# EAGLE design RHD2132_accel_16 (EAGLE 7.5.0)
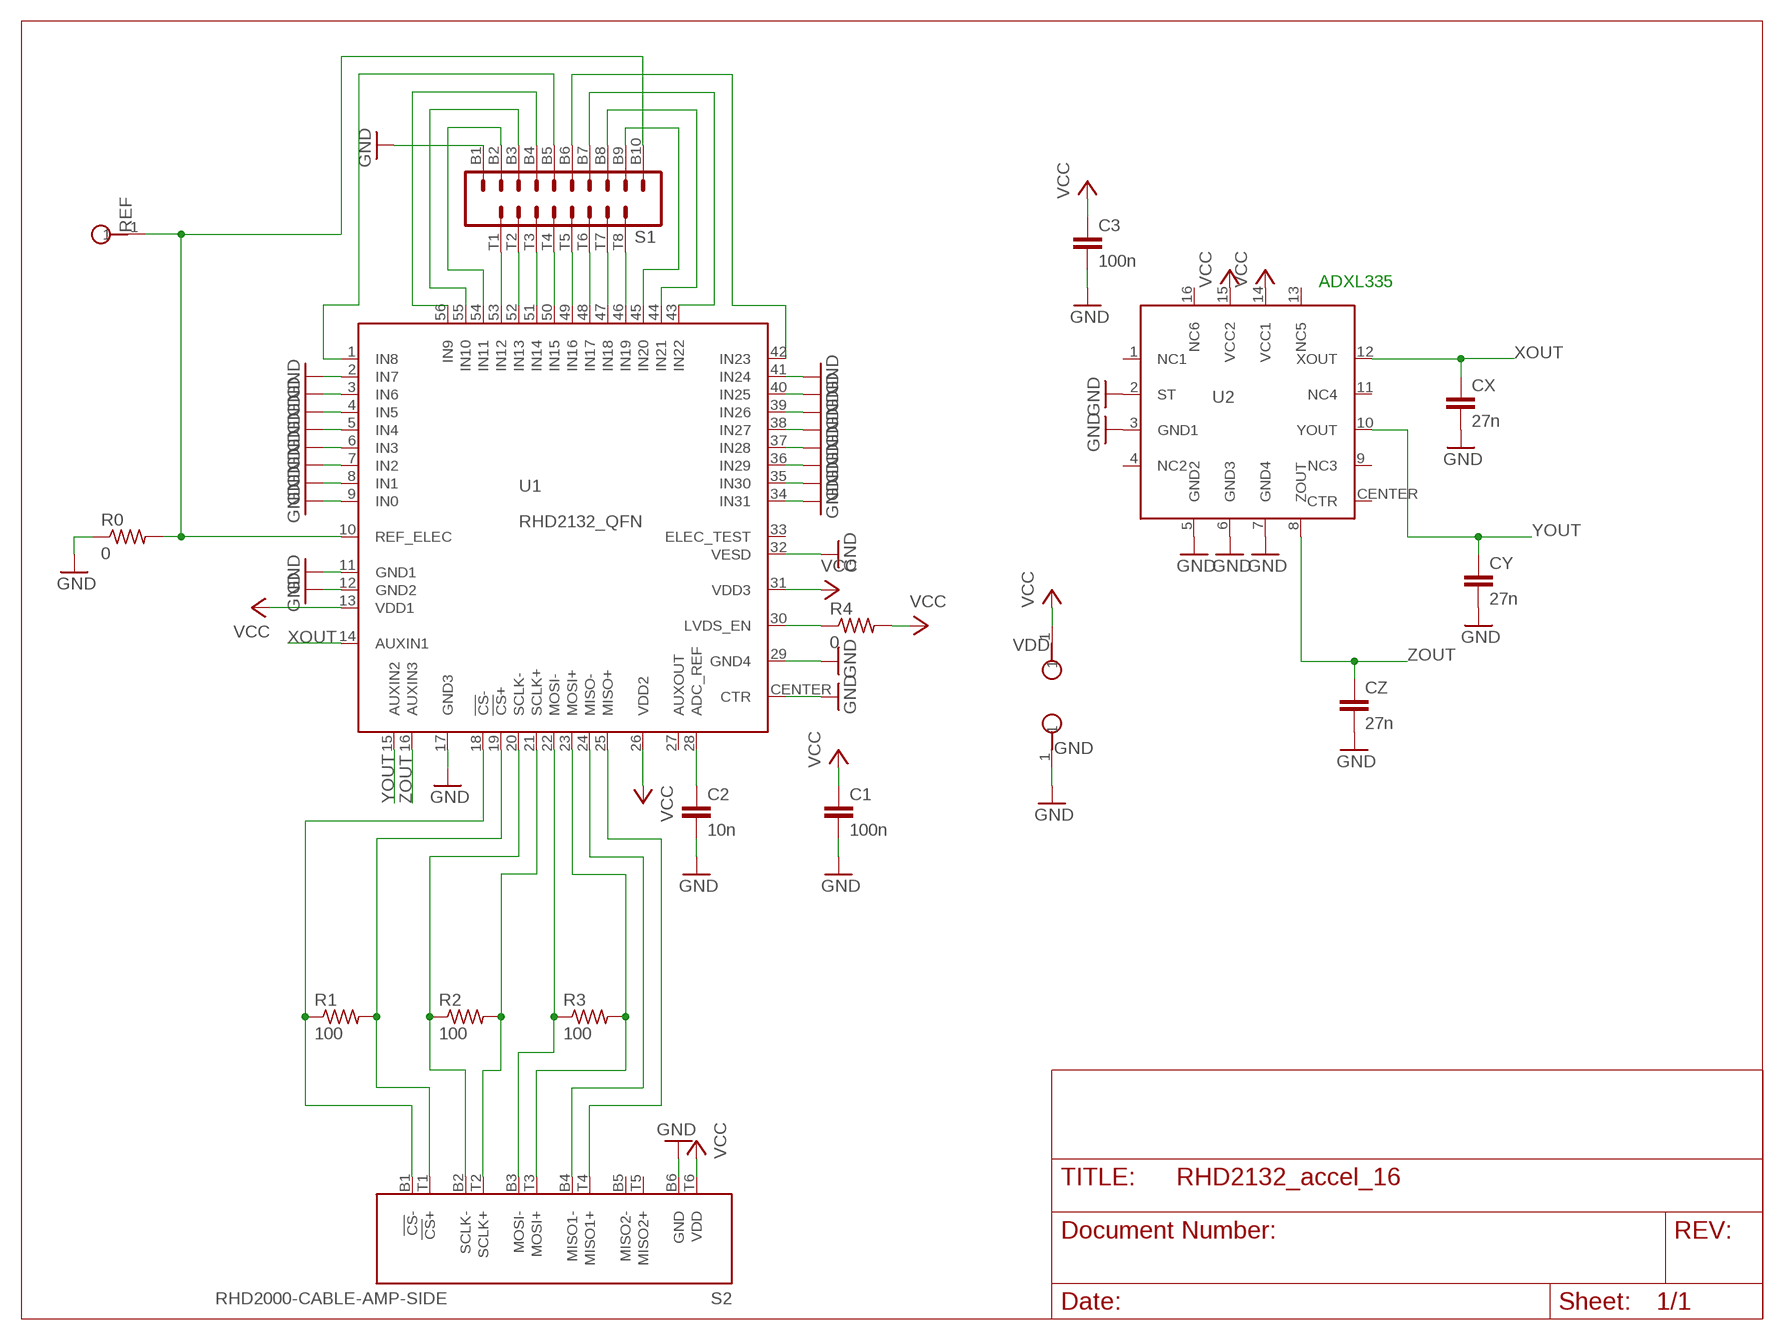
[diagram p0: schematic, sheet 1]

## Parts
C1  100n  C_0402  [0402]
C2  10n  C_0402  [0402]
C3  100n  C_0402  [0402]
CX  27n  C_0402  [0402]
CY  27n  C_0402  [0402]
CZ  27n  C_0402  [0402]
GND  TESTPOINT_SMALL  [TESTPOINT_SMALL]
R0  0  R_0402  [0402]
R1  100  R_0402  [0402]
R2  100  R_0402  [0402]
R3  100  R_0402  [0402]
R4  0  R_0402  [0402]
REF  TESTPOINT_SMALL  [TESTPOINT_SMALL]
S1  OMNETICS_A79041  [OMNETICS_A79041]
S2  RHD2000-CABLE-AMP-SIDE  [OMNETICS_PZN-12-AA]
U1  RHD2132_QFN  [QFN56_8_X_8_LARGE]
U2  ADXL335  [ADXL335]
VDD  TESTPOINT_SMALL  [TESTPOINT_SMALL]

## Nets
GND: C1.2 C2.2 C3.2 CX.2 CY.2 CZ.2 GND.1 R0.1 S1.B1 S2.B6(GND) U1.2(IN7) U1.3(IN6) U1.4(IN5) U1.5(IN4) U1.6(IN3) U1.7(IN2) U1.8(IN1) U1.9(IN0) U1.11(GND1) U1.12(GND2) U1.17(GND3) U1.29(GND4) U1.32(VESD) U1.34(IN31) U1.35(IN30) U1.36(IN29) U1.37(IN28) U1.38(IN27) U1.39(IN26) U1.40(IN25) U1.41(IN24) U1.CENTER(CTR) U2.2(ST) U2.3(GND1) U2.5(GND2) U2.6(GND3) U2.7(GND4)
N$1: R0.2 REF.1 S1.B10 U1.10(REF_ELEC)
N$2: S1.B5 U1.1(IN8)
N$3: S1.B4 U1.56(IN9)
N$4: S1.B3 U1.55(IN10)
N$5: S1.B2 U1.54(IN11)
N$6: S1.T1 U1.53(IN12)
N$7: S1.T2 U1.52(IN13)
N$8: S1.T3 U1.51(IN14)
N$9: S1.T4 U1.50(IN15)
N$10: S1.T5 U1.49(IN16)
N$11: R1.2 S2.T1(!CS!+) U1.19(!CS!+)
N$12: R4.1 U1.30(LVDS_EN)
N$13: S1.T6 U1.48(IN17)
N$14: S1.T7 U1.47(IN18)
N$15: S1.T8 U1.46(IN19)
N$16: S1.B9 U1.45(IN20)
N$17: S1.B8 U1.44(IN21)
N$18: S1.B7 U1.43(IN22)
N$19: S1.B6 U1.42(IN23)
N$21: R1.1 S2.B1(!CS!-) U1.18(!CS!-)
N$22: R2.1 S2.B2(SCLK-) U1.20(SCLK-)
N$37: R2.2 S2.T2(SCLK+) U1.21(SCLK+)
N$38: R3.1 S2.B3(MOSI-) U1.22(MOSI-)
N$39: R3.2 S2.T3(MOSI+) U1.23(MOSI+)
N$40: S2.B4(MISO1-) U1.24(MISO-)
N$41: S2.T4(MISO1+) U1.25(MISO+)
N$42: C2.1 U1.28(ADC_REF)
VCC: C1.1 C3.1 R4.2 S2.T6(VDD) U1.13(VDD1) U1.26(VDD2) U1.31(VDD3) U2.14(VCC1) U2.15(VCC2) VDD.1
XOUT: CX.1 U1.14(AUXIN1) U2.12(XOUT)
YOUT: CY.1 U1.15(AUXIN2) U2.10(YOUT)
ZOUT: CZ.1 U1.16(AUXIN3) U2.8(ZOUT)
Unconnected: S2.B5(MISO2-) S2.T5(MISO2+) U1.27(AUXOUT) U1.33(ELEC_TEST) U2.1(NC1) U2.4(NC2) U2.9(NC3) U2.11(NC4) U2.13(NC5) U2.16(NC6) U2.CENTER(CTR)

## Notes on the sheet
- ADXL335

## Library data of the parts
C1-C3 CX CY CZ = RHD2000_eval_board:C: Capacitor
GND REF VDD = RHD2000_eval_board:TESTPOINT: PCB Test Point
R0 R1-R4 = RHD2000_eval_board:R: Resistor
S1 = harrison:OMNETICS_A79041
S2 = RHD2000:RHD2000-CABLE-AMP-SIDE
U1 = INTAN:RHD2132: Intan Technologies RHD2132 chip
U2 = harrison:ADXL335

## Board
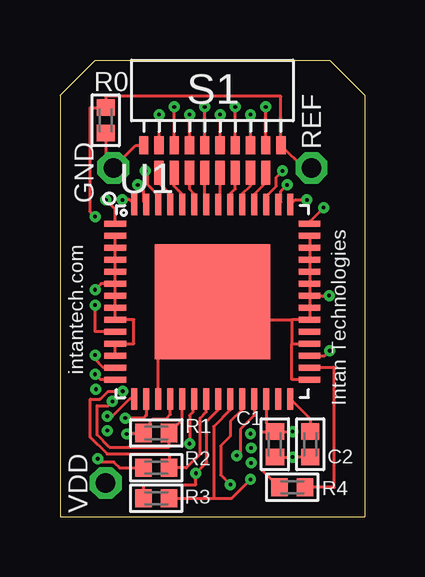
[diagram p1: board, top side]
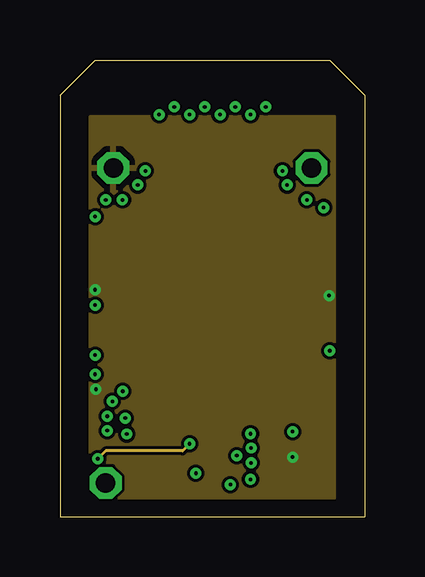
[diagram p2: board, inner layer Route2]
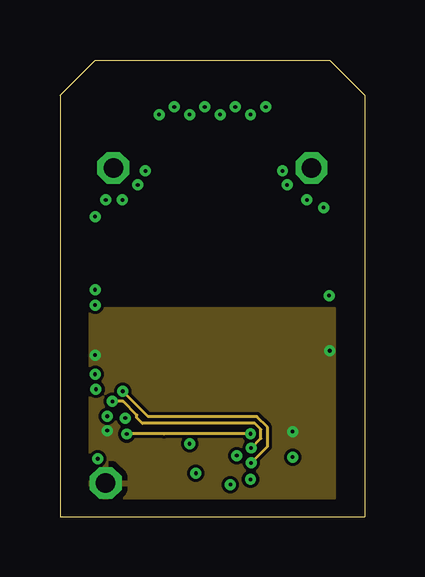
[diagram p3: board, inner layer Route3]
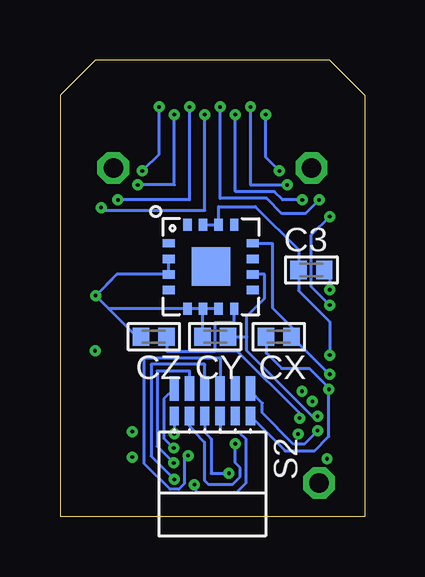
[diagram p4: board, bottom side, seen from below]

Size 12.7 x 19.02 mm. Coordinates in mm from the lower left corner, seen from the top.
Outline: 0,0 12.7,0 12.7,17.56 11.24,19.02 1.46,19.02 0,17.56 0,0
Copper layers (1*2+3*16): Top 0.035mm / dielectric 1.5mm / Route2 0.035mm / dielectric 0.15mm / Route3 0.035mm / dielectric 0.2mm / Bottom 0.035mm
Design rules "default *": minimum track width 5mil, minimum drill 6mil, track to track 5mil, track to pad 5mil, pad to pad 5mil, via to via 5mil, smd to smd 5mil, copper to edge 15mil, drill to drill 15mil, minimum pad ring 10mil, minimum via ring 6mil, stop-mask expansion 4mil, vias tented up to drill 0mil, thermal gap 10mil

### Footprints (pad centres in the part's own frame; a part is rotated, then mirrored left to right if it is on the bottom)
0402 = smd 0.686 x 0.762: 1 -0.533,0; 2 0.533,0
TESTPOINT_SMALL = drill 0.813 octagon: 1 0,0
OMNETICS_A79041 = smd 0.381 x 0.762: B1 -2.857,-1.016; B2 -2.223,-1.016; B3 -1.587,-1.016; B4 -0.953,-1.016; B5 -0.318,-1.016; B6 0.318,-1.016; B7 0.953,-1.016; B8 1.587,-1.016; B9 2.223,-1.016; B10 2.857,-1.016 | smd 0.381 x 1.016: T1 -2.223,-2.159; T2 -1.587,-2.159; T3 -0.953,-2.159; T4 -0.318,-2.159; T5 0.318,-2.159; T6 0.953,-2.159; T7 1.587,-2.159; T8 2.223,-2.159
OMNETICS_PZN-12-AA = smd 0.381 x 0.762: B1 1.587,-1.016; B2 0.953,-1.016; B3 0.318,-1.016; B4 -0.318,-1.016; B5 -0.953,-1.016; B6 -1.587,-1.016 | smd 0.381 x 1.016: T1 1.587,-2.159; T2 0.953,-2.159; T3 0.318,-2.159; T4 -0.318,-2.159; T5 -0.953,-2.159; T6 -1.587,-2.159
QFN56_8_X_8_LARGE = smd 0.9 x 0.25: 1 -4.05,3.25; 2 -4.05,2.75; 3 -4.05,2.25; 4 -4.05,1.75; 5 -4.05,1.25; 6 -4.05,0.75; 7 -4.05,0.25; 8 -4.05,-0.25; 9 -4.05,-0.75; 10 -4.05,-1.25; 11 -4.05,-1.75; 12 -4.05,-2.25; 13 -4.05,-2.75; 14 -4.05,-3.25; 29 4.05,-3.25; 30 4.05,-2.75; 31 4.05,-2.25; 32 4.05,-1.75; 33 4.05,-1.25; 34 4.05,-0.75; 35 4.05,-0.25; 36 4.05,0.25; 37 4.05,0.75; 38 4.05,1.25; 39 4.05,1.75; 40 4.05,2.25; 41 4.05,2.75; 42 4.05,3.25 | smd 0.25 x 0.9: 15 -3.25,-4.05; 16 -2.75,-4.05; 17 -2.25,-4.05; 18 -1.75,-4.05; 19 -1.25,-4.05; 20 -0.75,-4.05; 21 -0.25,-4.05; 22 0.25,-4.05; 23 0.75,-4.05; 24 1.25,-4.05; 25 1.75,-4.05; 26 2.25,-4.05; 27 2.75,-4.05; 28 3.25,-4.05; 43 3.25,4.05; 44 2.75,4.05; 45 2.25,4.05; 46 1.75,4.05; 47 1.25,4.05; 48 0.75,4.05; 49 0.25,4.05; 50 -0.25,4.05; 51 -0.75,4.05; 52 -1.25,4.05; 53 -1.75,4.05; 54 -2.25,4.05; 55 -2.75,4.05; 56 -3.25,4.05 | smd 4.8 x 4.8: CENTER 0,0
ADXL335 = smd 0.5 x 0.35: 1 -1.75,0.975; 2 -1.75,0.325; 3 -1.75,-0.325; 4 -1.75,-0.975; 9 1.75,-0.975; 10 1.75,-0.325; 11 1.75,0.325; 12 1.75,0.975 | smd 0.35 x 0.5: 5 -0.975,-1.75; 6 -0.325,-1.75; 7 0.325,-1.75; 8 0.975,-1.75; 13 0.975,1.75; 14 0.325,1.75; 15 -0.325,1.75; 16 -0.975,1.75 | smd 1.6 x 1.6: CENTER 0,0

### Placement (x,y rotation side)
C1  8.95,3.01 270 top
C2  10.43,3.01 270 top
C3  2.22,10.27 0 bottom
CX  3.58,7.49 180 bottom
CY  6.24,7.49 180 bottom
CZ  8.79,7.49 180 bottom
GND  2.22,14.53 90 top
R0  1.91,16.51 90 top
R1  4.01,3.48 0 top
R2  4.01,2.03 0 top
R3  4.01,0.76 0 top
R4  9.68,1.22 180 top
REF  10.48,14.53 270 top
S1  6.35,16.48 0 top
S2  6.35,3.17 180 bottom
U1  6.35,8.95 0 top
U2  6.41,10.41 0 bottom
VDD  1.91,1.4 0 top

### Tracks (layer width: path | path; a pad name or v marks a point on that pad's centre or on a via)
GND  (via drill 0.15)
  Top 0.127: U1.CENTER 6.35,9.38 | 4.1,9.13 U1.CENTER | U1.12 U1.11 3.07,7.2 3.07,8.2 U1.9 U1.8 U1.7 U1.6 | U1.6 1.72,9.7 v1.46,9.45 | U1.6 U1.5 U1.4 U1.3 U1.2 | U1.41 U1.40 U1.39 U1.38 U1.37 U1.36 | 9.66,8.2 U1.34 U1.35 U1.36 | 9.66,8.2 9.66,7.2 | 9.66,7.2 U1.32 | U1.29 9.66,5.7 9.66,7.2 | U1.CENTER 7.1,8.2 9.66,8.2 | C2.2 v9.69,2.48 C1.2 | U1.17 4.1,6.7 U1.CENTER | U1.36 v11.21,9.2 v11.21,9.21 | R0.1 1.91,14.85 GND.1 3.16,15.47 S1.B1
  Route2 0.127: v1.46,9.45 1.52,9.38 | v9.69,2.48 9.69,2.45 | v11.21,9.21 11.21,9.11
  Bottom 0.127: U2.2 U2.3 10.33,10.09 v11.21,9.21 | C3.2 arc90 1.46,10.05 v1.46,9.45 | S2.B6 3.31,2.74 2.1,2.74 1.5,3.34 v1.5,5.31 1.5,5.36 2.31,6.17 3.47,6.17 4.12,6.82 CX.2 | 6.77,8.44 U2.6 U2.7 | 10.52,9.9 v11.21,9.21 | 6.77,8.44 CY.2 | 6.77,8.44 6.77,8.66 U2.5 10.67,8.66 v11.21,9.21 | CZ.2 9.5,7.49 v11.21,9.21
  pour Route2: 1.27,0.76 1.27,16.69 11.43,16.69 11.43,0.76
N$1  (via drill 0.15)
  Top 0.127: v1.46,12.5 1.27,12.69 1.27,17.04 R0.2 1.91,17.51 9.21,17.51 S1.B10 10.15,14.53 REF.1 10.35,14.53 | U1.10 1.46,7.7 v1.46,8.81
  Bottom 0.127: v1.46,12.5 2.22,11.73 2.22,9.58 v1.46,8.81
N$2  (via drill 0.15)
  Top 0.127: U1.1 2.3,12.8 v1.91,13.2 | S1.B5 v6.03,17.07
  Bottom 0.127: v1.91,13.2 2.48,12.62 3.45,12.62 4.09,13.26 6.03,13.26 v6.03,17.07
N$3  (via drill 0.15)
  Top 0.127: U1.56 2.91,13.2 v2.6,13.2 | S1.B4 v5.4,16.75
  Bottom 0.127: v2.6,13.2 3.43,13.2 3.77,13.54 5.4,13.54 v5.4,16.75
N$4  (via drill 0.15)
  Top 0.127: U1.55 3.48,13.12 3.48,13.58 v3.24,13.82 | S1.B3 v4.76,17.07
  Bottom 0.127: v3.24,13.82 4.76,13.82 v4.76,17.07
N$5  (via drill 0.15)
  Top 0.127: S1.B2 v4.13,16.75 | v3.56,14.4 3.66,14.3 3.66,13.82 4.1,13.38 U1.54
  Bottom 0.127: v3.56,14.4 4.13,14.97 v4.13,16.75
N$6
  Top 0.127: U1.53 4.6,13.42 4.13,13.89 S1.T1
N$7
  Top 0.127: U1.52 5.1,13.43 4.76,13.77 S1.T2
N$8
  Top 0.127: U1.51 5.6,13.44 5.4,13.64 S1.T3
N$9
  Top 0.127: U1.50 6.03,13.07 S1.T4
N$10
  Top 0.127: U1.49 6.67,13.07 S1.T5
N$11  (via drill 0.15)
  Top 0.127: v2.18,4.8 2.01,4.62 1.55,4.62 1.55,3.4 2.06,2.9 4.55,2.9 R1.2 5.1,4.03 U1.19
  Route3 0.127: v7.96,2.86 8.37,3.26 8.37,3.63 8.12,3.89 3.43,3.89 3.2,4.12 3.2,4.23 2.63,4.8 v2.18,4.8
  Bottom 0.127: S2.T1 8.37,4.9 8.37,3.26 v7.96,2.86
N$12
  Top 0.127: U1.30 11.43,6.2 11.43,1.22 R4.1
N$13
  Top 0.127: U1.48 7.1,13.45 7.3,13.65 S1.T6
N$14
  Top 0.127: U1.47 7.6,13.46 7.94,13.79 S1.T7
N$15
  Top 0.127: U1.46 8.1,13.43 8.57,13.91 S1.T8
N$16  (via drill 0.15)
  Top 0.127: v9.27,14.4 9.02,14.15 9.02,13.77 8.6,13.35 U1.45 | S1.B9 v8.57,17.07
  Bottom 0.127: v9.27,14.4 8.57,15.1 v8.57,17.07
N$17  (via drill 0.15)
  Top 0.127: U1.44 9.21,13.11 9.21,13.56 v9.46,13.82 | S1.B8 v7.94,16.75
  Bottom 0.127: v9.46,13.82 7.94,13.82 v7.94,16.75
N$18  (via drill 0.15)
  Top 0.127: 10.29,13.18 v10.29,13.2 9.79,13.2 U1.43 | S1.B7 v7.3,17.07
  Bottom 0.127: v10.29,13.2 7.3,13.2 v7.3,17.07
N$19  (via drill 0.15)
  Top 0.127: U1.42 10.4,12.29 v10.99,12.88 | S1.B6 v6.67,16.75
  Bottom 0.127: v10.99,12.88 10.86,12.75 6.67,12.75 v6.67,16.75
N$21  (via drill 0.15)
  Top 0.127: U1.18 4.6,4.25 4.41,4.06 3.85,4.06 3.75,3.96 3.75,3.75 R1.1 | 3.48,3.66 R1.1 | R1.1 3.44,3.44 v2.78,3.44
  Route3 0.127: v2.78,3.44 4.33,3.44 4.34,3.45 v7.94,3.45
  Bottom 0.127: S2.B1 v7.94,3.45
N$22  (via drill 0.15)
  Top 0.127: U1.20 5.54,4.84 5.54,4.36 5.4,4.22 v5.4,3.04 | v1.57,2.41 1.71,2.27 2.25,2.27 2.49,2.03 R2.1
  Route2 0.127: v1.57,2.41 1.91,2.74 5.11,2.74 v5.4,3.04
  Bottom 0.127: v5.4,3.04 5.4,2.23 5.19,2.03 5.19,1.66 5.52,1.33 6.5,1.33 6.68,1.51 6.68,3.1 7.11,3.53 7.11,3.58 7.3,3.77 S2.B2
N$37  (via drill 0.15)
  Top 0.127: U1.21 6.1,4.36 5.84,4.1 5.84,2.6 5.27,2.03 R2.2 4.55,2.62 1.97,2.62 1.27,3.31 1.27,4.89 1.68,4.89 2.01,5.22 v2.62,5.22
  Route3 0.127: v7.96,2.23 8.65,2.92 8.65,3.72 8.2,4.17 3.67,4.17 v2.62,5.22
  Bottom 0.127: S2.T2 7.3,6.06 8.65,6.06 8.65,2.92 v7.96,2.23
N$38  (via drill 0.15)
  Top 0.127: R3.1 3.48,1.33 5.66,1.33 v5.66,1.8 6.12,2.26 6.12,3.98 6.6,4.45 U1.22
  Bottom 0.127: S2.B3 6.67,3.5 6.4,3.24 6.4,1.8 v5.66,1.8
N$39  (via drill 0.15)
  Top 0.127: 7.04,4.9 U1.23 7.1,4.45 6.4,3.75 6.4,0.76 | R3.2 6.4,0.76 | 6.4,0.76 7.15,0.76 v7.94,1.55
  Bottom 0.127: S2.T3 6.67,6.34 8.9,6.34 8.9,2.52 v7.94,1.55
N$40  (via drill 0.15)
  Top 0.127: U1.24 7.59,4.46 7.1,3.96 7.1,3.35 6.69,2.95 6.69,1.74 v7.1,1.33 6.97,1.46
  Bottom 0.127: S2.B4 6.03,3.52 5.25,3.52 4.94,3.21 4.94,1.41 5.36,0.99 6.95,0.99 7.11,1.16 v7.1,1.33
N$41  (via drill 0.15)
  Top 0.127: U1.25 8.1,4.21 7.52,3.63 7.52,2.69 v7.37,2.54
  Bottom 0.127: v7.37,2.54 7.52,2.39 7.52,1.37 7.76,1.13 8.12,1.13 9.18,2.2 9.18,6.62 6.03,6.62 S2.T4
N$42
  Top 0.127: U1.28 10.43,4.08 C2.1
VCC  (via drill 0.15)
  Top 0.127: U1.31 11.03,6.7 v11.24,6.91 | U1.26 8.6,3.9 C1.1 | C1.1 v9.69,3.54 | C1.1 8.38,3.54 8.38,1.98 R4.2 9.09,1.32 | U1.13 1.81,6.2 1.46,6.55 v1.46,6.73
  Route3 0.127: v11.24,6.91 11.24,6.78 | v9.69,3.54 9.69,3.5
  Bottom 0.127: v1.46,6.73 1.46,8.12 2.76,9.41 C3.1 2.76,11.11 4.56,12.92 6.09,12.92 U2.14 U2.15 | v1.97,3.58 2.53,3.02 2.97,3.02 4.27,4.32 4.27,4.72 4.76,5.22 S2.T6
  pour Route3: 1.27,0.76 1.27,8.69 11.43,8.69 11.43,0.76
XOUT  (via drill 0.15)
  Top 0.127: U1.14 1.69,5.7 v1.46,5.93
  Bottom 0.127: U2.12 3.85,11.39 3.85,8.7 3.05,7.9 CX.1 1.49,5.93 v1.46,5.93
YOUT  (via drill 0.15)
  Top 0.127: U1.15 2.91,4.9 2.18,4.18 v1.97,4.18
  Bottom 0.127: CY.1 4.92,7.49 | 4.92,7.49 4.92,8.36 4.18,9.09 4.18,10.09 U2.10 | v1.97,4.18 2.18,4.18 4.92,6.91 4.92,7.49
ZOUT  (via drill 0.15)
  Top 0.127: U1.16 3.6,4.22 3.49,4.1 v2.72,4.1
  Bottom 0.127: CZ.1 8.26,6.9 6.24,6.9 | 6.24,6.9 6.24,8.09 5.44,8.09 U2.8 | 6.24,6.9 5.31,6.9 2.72,4.3 v2.72,4.1

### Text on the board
tPlace: intantech.com | Intan Technologies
